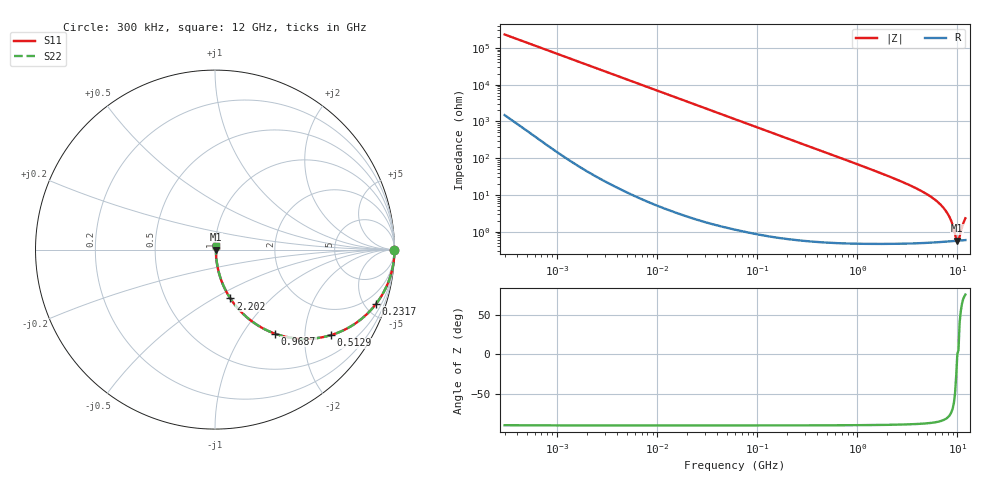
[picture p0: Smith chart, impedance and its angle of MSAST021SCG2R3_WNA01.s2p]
! MSAST021SCG2R3_WNA01  S-PARAMETER MODEL  ( General Type )
! Model Generated by TAIYO YUDEN Corporation (http://www.ty-top.com)
! Version 2.0
! TAIYO YUDEN Control No. 181101
! Copyright(c) 2015 TAIYO YUDEN CO.,LTD. All Rights Reserved.
! Product Description (link to TY-COMPAS)
! https://ds.yuden.co.jp/TYCOMPAS/or/detail?pn=MSAST021SCG2R3BWNA01&u=M
! Products Name : Multilayer Ceramic Capacitors
! Characteristics :
!  Capacitance : 2.3 pF , Rated Voltage : 25V , TCC : CG / C0G
!  Case Size : 0.25 x 0.125 / 0.0098 x 0.0049 [mm/inch] , Thickness : 0.125 / 0.0049 [mm/inch]
!  (Conditions: Temperature = 25 degC , DC Bias Current/Voltage = 0A / 0V)
! External Node Assignments :
!  1  o---| |---o  2
! GND o---------o GND
! Frequency Range : 0.3MHz  -  12000MHz  [ 401 STEP ]
# MHz S RI R 50
! Freq[MHz].  S11 Real  S11 Imag  S21 Real  S21 Imag  S12 Real  S12 Imag  S22 Real  S22 Imag
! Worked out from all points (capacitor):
!   401 points, 300 kHz to 12 GHz, reference 50 ohm
!   read as one part in series: C = 2.3 pF near 316.3 kHz
!   lowest |Z| = 569 mohm at 9.969 GHz (marker M1)
!   series resonance near 9.969 GHz, so ESL is about 110 pH
!   S11 on the Smith chart (normalised r, x): 300 kHz: open; 231.7 MHz: 1.01, -5.97; 512.9 MHz: 1.01, -2.69; 968.7 MHz: 1.01, -1.42; 2.202 GHz: 1.01, -0.60; 12 GHz: 1.01, +0.04
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0.3  1 -0.000434  2.97e-06 0.000434  2.97e-06 0.000434  1 -0.000434
1.769972  1 -0.00256  1e-05 0.00256  1e-05 0.00256  1 -0.00256
10.44266  0.9998 -0.0151  0.000239 0.0151  0.000239 0.0151  0.9998 -0.0151
60  0.9925 -0.086  0.00755 0.086  0.00755 0.086  0.9925 -0.086
119.4772  0.9708 -0.1676  0.0292 0.1676  0.0292 0.1676  0.9708 -0.1676
231.6935  0.8986 -0.3008  0.1014 0.3008  0.1014 0.3008  0.8986 -0.3008
353.9943  0.7915 -0.4049  0.2085 0.4049  0.2085 0.4049  0.7915 -0.4049
512.9422  0.6436 -0.4771  0.3564 0.4771  0.3564 0.4771  0.6436 -0.4771
968.706  0.3346 -0.4685  0.6654 0.4685  0.6654 0.4685  0.3346 -0.4685
1403.667  0.1916 -0.3887  0.8084 0.3887  0.8084 0.3887  0.1916 -0.3887
2088.533  0.0946 -0.2853  0.9054 0.2853  0.9054 0.2853  0.0946 -0.2853
2202.174  0.0855 -0.2719  0.9145 0.2719  0.9145 0.2719  0.0855 -0.2719
4270.516  0.0217 -0.1285  0.9783 0.1285  0.9783 0.1285  0.0217 -0.1285
6524.734  0.00873 -0.0593  0.9913 0.0593  0.9913 0.0593  0.00873 -0.0593
7254.098  0.00722 -0.0438  0.9928 0.0438  0.9928 0.0438  0.00722 -0.0438
8064.993  0.00624 -0.0287  0.9938 0.0287  0.9938 0.0287  0.00624 -0.0287
8732.115  0.00581 -0.0176  0.9942 0.0176  0.9942 0.0176  0.00581 -0.0176
9708.23  0.00564 -0.00293  0.9944 0.00293  0.9944 0.00293  0.00564 -0.00293
9968.853  0.00566 1.55e-06  0.9943 -1.55e-06  0.9943 -1.55e-06  0.00566 1.55e-06
10511.28  0.00575 0.00478  0.9942 -0.00478  0.9942 -0.00478  0.00575 0.00478
11380.75  0.00606 0.0151  0.9939 -0.0151  0.9939 -0.0151  0.00606 0.0151
12000  0.00639 0.0221  0.9936 -0.0221  0.9936 -0.0221  0.00639 0.0221
